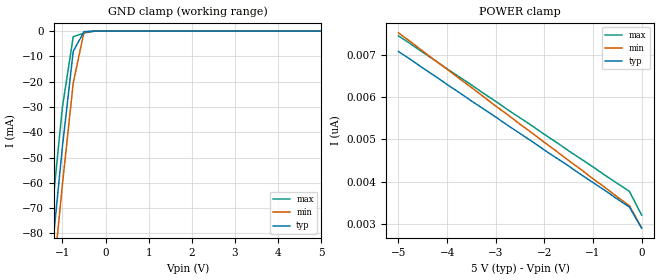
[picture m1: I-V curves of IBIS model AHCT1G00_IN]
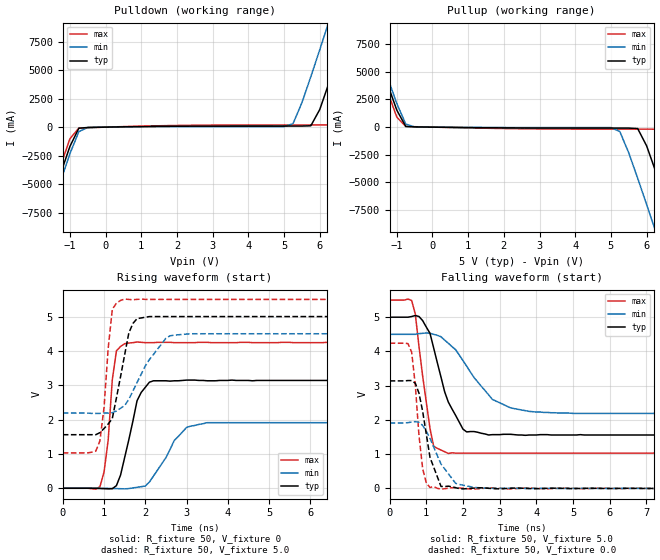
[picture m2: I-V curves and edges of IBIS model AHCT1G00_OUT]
| TEXAS INSTRUMENTS INCORPORATED
| Standard Linear and Logic Group
| IBIS Model of SN74AHCT1G00
| SINGLE 2-INPUT POSITIVE-NAND GATE
| SOT 5-pin (DCK) and SOT 5-pin (DBV) Package
[IBIS Ver]   3.2
[Comment Char]  |_char
[File Name]   ahct1g00.ibs
[File Rev]   2.0 J_die
[Date]   May 24, 2000
[Source]   Data created from HSPICE simulations at TI-SLL.
[Notes]   The following is an IBIS list for the AHCT1G00.
|   Please contact sllibis@ti.com with questions and
|   comments concerning SLL IBIS models.
[Disclaimer] Property of Texas Instruments Incorporated.  Unauthorized
   reproduction and/or distribution is strictly prohibited.
   This product is protected under copyright law.
   Created 2000, (C) Copyright 2000, Texas Instruments Inc.,
   All Rights Reserved.
   UNLESS THERE IS A SIGNED, WRITTEN AGREEMENT TO THE
   CONTRARY, TEXAS INSTRUMENTS () IS PROVIDING THE IBIS
   MODELS  AND WITHOUT ANY WARRANTY, EXPRESSED OR
   IMPLIED.  TI assumes no liability for:
   1) the accuracy of the IBIS models provided to your
   company;
   2) the proper functioning of these IBIS Models in your
   design or for any resulting applications; or
   3) infringement of patents, copyrights or intellectual
   property rights resulting from your use of these IBIS
   models.
   TI provides IBIS Models as a service to our customers.
   You and your company shall not distribute, sell or give
   these models to anyone else without prior written
   permission from TI.
   TI reserves the right to make changes to our products or
   to discontinue any semiconductor product or service
   without notice, and advises our customers to obtain the
   latest version of relevant information to verify, before
   placing orders, that the information being relied on is
   current.
   Please be aware that your receipt and use of the IBIS
   information provided shall serve as acceptance of these
   terms and conditions.  If you do not accept these terms,
   you should return or destroy the IBIS models and any
   other accompanying information immediately.
|   Component AHCT1G00_DCK
[Component]   AHCT1G00_DCK
[Manufacturer]  Texas Instruments, Inc.
[Package]
|   typ   min   max
R_pkg   0.020   0.017   0.025
L_pkg   0.998nH   0.881nH   1.069nH
C_pkg   0.146pF   0.118pF   0.205pF
[Pin]   signal_name   model_name   R_pin   L_pin   C_pin
1   A   AHCT1G00_IN   0.019   1.069nH   0.162pF
2   B   AHCT1G00_IN   0.018   0.881nH   0.121pF
3   GND   GND   0.017   1.031nH   0.205pF
4   Y   AHCT1G00_OUT   0.020   0.960nH   0.124pF
5   VCC   POWER   0.025   1.049nH   0.118pF
|   Component AHCT1G00_DBV
[Component]   AHCT1G00_DBV
[Manufacturer]  Texas Instruments, Inc.
[Package]
|   typ   min   max
R_pkg   0.025   0.021   0.029
L_pkg   1.529nH   1.312nH   1.906nH
C_pkg   0.156pF   0.110pF   0.240pF
[Pin]   signal_name   model_name   R_pin   L_pin   C_pin
1   A   AHCT1G00_IN   0.021   1.511nH   0.144pF
2   B   AHCT1G00_IN   0.023   1.312nH   0.138pF
3   GND   GND   0.029   1.906nH   0.240pF
4   Y   AHCT1G00_OUT   0.026   1.541nH   0.150pF
5   VCC   POWER   0.025   1.374nH   0.110pF
| Models and submodels in the file (2): AHCT1G00_IN (Input), AHCT1G00_OUT (Output)
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|   Model AHCT1G00_IN
[Model]   AHCT1G00_IN
Model_type  Input
Polarity   Inverting
Vinl = 0.8
Vinh = 2.0
| variable   typ   min   max
C_comp   1.24pf   0.93pf   1.55pf
[Temperature Range]   25   85   -40
[Voltage Range]   5.0   4.5   5.5
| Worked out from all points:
|   GND clamp passes 1 mA (typ) near -0.52 V on its own axis
[GND Clamp]
|   Voltage   I(typ)   I(min)   I(max)
-5V       -773mA     -786mA     -758mA
-1.5V     -133mA     -148mA     -117mA
-1.25V    -88.7mA    -104mA     -72.7mA
-1V       -45.6mA    -60.5mA    -30mA
-750mV    -7.99mA    -20.5mA    -2.23mA
-500mV    -233uA     -353uA     -759uA
-250mV    -2.63nA    -182nA     -26.9uA
5V        2.9nA      3.64nA     2.54nA
[POWER Clamp]
|   Voltage   I(typ)   I(min)   I(max)
-5V       7.08nA     7.52nA     7.45nA
-1.5V     4.37nA     4.5nA      4.73nA
-250mV    3.4nA      3.43nA     3.77nA
0V        2.9nA      2.91nA     3.21nA
|   Model AHCT1G00_OUT
[Model]   AHCT1G00_OUT
Model_type  Output
Polarity   Inverting
Vmeas = 2.50v
Cref = 15pf
| variable   typ   min   max
C_comp   3.12pf   2.34pf   3.90pf
[Temperature Range]   25   85   -40
[Voltage Range]   5.0   4.5   5.5
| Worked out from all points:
|   slope of the pulldown table from 0 to 0.75 V, typ, clamps not added: 18.8 ohm
|   slope of the pullup table from 0 to 0.75 V, typ, clamps not added: 25.3 ohm
|   rising waveform, R_fixture 50, V_fixture 0: 20-80 % time 346ps typ, 601ps min, 187ps max; typ from 0 V to 3.14 V
|   falling waveform, R_fixture 50, V_fixture 5.0: 20-80 % time 587ps typ, 952ps min, 326ps max; typ from 5 V to 1.56 V
|   rising waveform, R_fixture 50, V_fixture 5.0: 20-80 % time 331ps typ, 660ps min, 191ps max; typ from 1.56 V to 5 V
|   falling waveform, R_fixture 50, V_fixture 0.0: 20-80 % time 347ps typ, 566ps min, 211ps max; typ from 3.14 V to 0 V
[Pulldown]
|   Voltage   I(typ)   I(min)   I(max)
-5V       -40.9A     -41.4A     -40.3A
-1.75V    -8.76A     -9.39A     -8.09A
-1V       -1.69A     -2.33A     -1.02A
-750mV    -95.5mA    -395mA     -80.6mA
5.25V     93.4mA     298mA      192mA
5.75V     116mA      4.42A      192mA
6.25V     3.8A       9.19A      193mA
6.5V      6.17A      11.6A      931mA
6.75V     8.59A      14.1A      3.15A
7.25V     13.5A      19A        7.96A
7.5V      15.9A      21.4A      10.4A
10V       40.7A      46.2A      35.2A
[Pullup]
|   Voltage   I(typ)   I(min)   I(max)
-5V       40.7A      41.2A      40.1A
-2V       11A        11.6A      10.4A
-1.75V    8.59A      9.19A      7.96A
-1V       1.54A      2.14A      907mA
-750mV    63.6mA     284mA      62.5mA
5.25V     -84.4mA    -401mA     -178mA
5.75V     -130mA     -4.62A     -178mA
6.25V     -3.97A     -9.39A     -187mA
6.75V     -8.76A     -14.3A     -3.28A
7.25V     -13.6A     -19.2A     -8.09A
7.5V      -16.1A     -21.6A     -10.5A
10V       -40.9A     -46.4A     -35.3A
[Ramp]
| variable   typ   min   max
dV/dt_r   1.91E+00/3.26E-10   1.18E+00/5.35E-10   2.56E+00/1.88E-10
dV/dt_f   2.10E+00/5.54E-10   1.41E+00/9.87E-10   2.74E+00/2.70E-10
R_load = 50
[Rising Waveform]
R_fixture = 50
V_fixture = 0
|   Time   V(typ)   V(min)   V(max)
0s        0V         0V         0V
900ps     -6.94mV    639uV      45.3mV
1.1ns     -16.6mV    -3.27mV    1.4V
1.3ns     76.8mV     -8.59mV    4V
1.6ns     1.41V      -8.47mV    4.23V
1.8ns     2.55V      27.8mV     4.26V
2.1ns     3.09V      183mV      4.24V
3ns       3.15V      1.77V      4.24V
3.5ns     3.13V      1.91V      4.25V
25ns      3.14V      1.91V      4.24V
[Falling Waveform]
R_fixture = 50
V_fixture = 5.0
V_fixture_min = 4.5
V_fixture_max = 5.5
|   Time   V(typ)   V(min)   V(max)
0s        5V         4.5V       5.5V
600ps     5.02V      4.5V       5.49V
700ps     5.05V      4.5V       5.09V
900ps     4.9V       4.53V      3.28V
1.2ns     4.1V       4.5V       1.23V
1.6ns     2.52V      4.24V      1.02V
2.1ns     1.65V      3.57V      1.03V
2.8ns     1.57V      2.6V       1.03V
4ns       1.56V      2.23V      1.03V
25ns      1.56V      2.19V      1.03V
[Rising Waveform]
R_fixture = 50
V_fixture = 5.0
V_fixture_min = 4.5
V_fixture_max = 5.5
|   Time   V(typ)   V(min)   V(max)
0s        1.56V      2.19V      1.03V
800ps     1.56V      2.18V      1.08V
900ps     1.62V      2.18V      1.38V
1ns       1.74V      2.19V      2.35V
1.2ns     2.03V      2.2V       5.21V
1.5ns     3.89V      2.41V      5.51V
1.8ns     4.94V      3.08V      5.5V
2.5ns     5V         4.37V      5.5V
3.1ns     5V         4.5V       5.5V
25ns      5V         4.5V       5.5V
[Falling Waveform]
R_fixture = 50
V_fixture = 0.0
|   Time   V(typ)   V(min)   V(max)
0s        3.14V      1.91V      4.24V
600ps     3.15V      1.94V      3.98V
700ps     3.07V      1.95V      3.01V
800ps     2.78V      1.93V      1.54V
900ps     2.25V      1.84V      573mV
1.1ns     904mV      1.46V      25.8mV
1.4ns     57.2mV     711mV      -22.2mV
1.8ns     19.9mV     147mV      23.6mV
2.4ns     16.7mV     21.9mV     -11.3mV
25ns      0V         0V         0V
